(* Logix 5000 AddOnInstructionDefinition export CFW900_2070; software revision 20.06 *)

ADD_ON_INSTRUCTION CFW900_2070   (* revision 1.0, ExecutePrescan *)
// 20/70 CIP Basic Speed
// AOI
// Help:
// Drive setup as follows:
// C9.5.1 = 20/70
// C4.1.1 - Remote 2
// C4.2.2.1 - Ethernet
// C4.2.2.2 - Ethernet
// C4.2.2.3 - Ethernet
// C4.2.2.4 - Ethernet
// C4.3.1.2.1 - Keypad
// C4.3.1.2.2 - Ethernet
VAR_INPUT
   ConnectionFaulted : BOOL; {required}   // From CFW900
END_VAR
VAR_IN_OUT
   InputData : INT[2]; {required}   // Input Assembly From CFW900
   OutputData : INT[2]; {required}   // Output Assembly To CFW900
END_VAR
VAR_INPUT
   Run : BOOL; {visible}   // 1 = Run 0 = Stop
   Fault_Reset : BOOL; {visible}   // 1 = Clear fault 0 = no action
   cfg_FailToStartDelay : DINT; {visible}   // Time in seconds before faulting on fail to start if vfd doesn't start on command (0 to disable)
   cfg_FailToStopDelay : DINT; {visible}   // Time in seconds before faulting on fail to stop if vfd doesn't stop on command (0 to disable)
END_VAR
VAR_OUTPUT
   Connection_Ready : BOOL; {access Read Only, visible}   // 1 = Connection to VFD is established to PLC
   Connection_Faulted : BOOL; {access Read Only, visible}   // Connection_Faulted Status Bit
   Running : BOOL; {access Read Only, visible}   // 1 = CFW900 Running 0 = CFW900 Stopped
   Faulted : BOOL; {access Read Only, visible}   // AOI Faulted Connection fault or failed to start / stop as well as VFD faults
END_VAR
VAR_INPUT
   Speed_Reference : INT; {required}   // Speed Setpoint (RPM) Negative speed will reverse direction
END_VAR
VAR_OUTPUT
   RealSpeed : INT; {access Read Only, visible}   // Current Speed (RPM)
END_VAR
VAR
   FailToStart : TIMER; {access None}
   FailToStop : TIMER;
   Wrk_Run1 : BOOL; {access None}
END_VAR

ROUTINE Logic   (* ladder *)
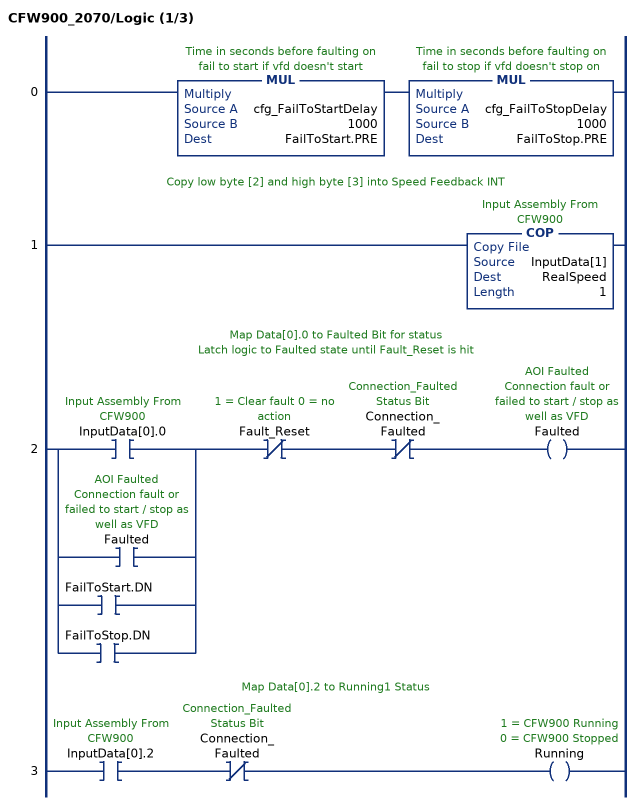
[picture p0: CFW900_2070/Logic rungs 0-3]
   0: MUL(cfg_FailToStartDelay,1000,FailToStart.PRE)MUL(cfg_FailToStopDelay,1000,FailToStop.PRE);
   // Copy low byte [2] and high byte [3] into Speed Feedback INT
   1: COP(InputData[1],RealSpeed,1);
   // Map Data[0].0 to Faulted Bit for status
   // Latch logic to Faulted state until Fault_Reset is hit
   2: [XIC(InputData[0].0) ,XIC(Faulted) ,XIC(FailToStart.DN) ,XIC(FailToStop.DN) ]XIO(Fault_Reset)XIO(Connection_Faulted)OTE(Faulted);
   // Map Data[0].2 to Running1 Status
   3: XIC(InputData[0].2)XIO(Connection_Faulted)OTE(Running);
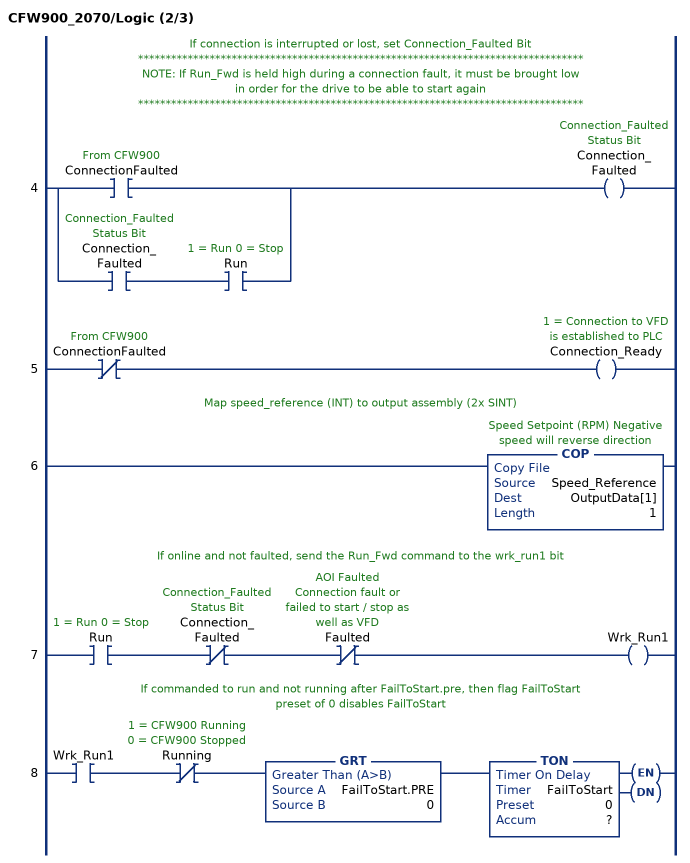
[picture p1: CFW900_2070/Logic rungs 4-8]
   // If connection is interrupted or lost, set Connection_Faulted Bit
   // *********************************************************************************
   // NOTE: If Run_Fwd is held high during a connection fault, it must be brought low
   // in order for the drive to be able to start again
   // *********************************************************************************
   4: [XIC(ConnectionFaulted) ,XIC(Connection_Faulted) XIC(Run) ]OTE(Connection_Faulted);
   5: XIO(ConnectionFaulted)OTE(Connection_Ready);
   // Map speed_reference (INT) to output assembly (2x SINT)
   6: COP(Speed_Reference,OutputData[1],1);
   // If online and not faulted, send the Run_Fwd command to the wrk_run1 bit
   7: XIC(Run)XIO(Connection_Faulted)XIO(Faulted)OTE(Wrk_Run1);
   // If commanded to run and not running after FailToStart.pre, then flag FailToStart
   // preset of 0 disables FailToStart
   8: XIC(Wrk_Run1)XIO(Running)GRT(FailToStart.PRE,0)TON(FailToStart,?,?);
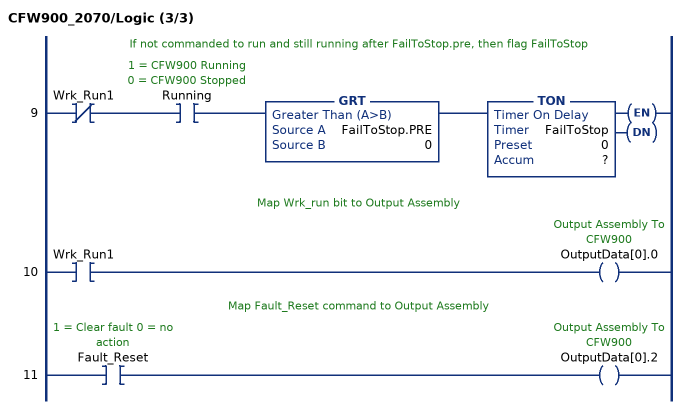
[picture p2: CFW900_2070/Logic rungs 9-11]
   // If not commanded to run and still running after FailToStop.pre, then flag FailToStop
   9: XIO(Wrk_Run1)XIC(Running)GRT(FailToStop.PRE,0)TON(FailToStop,?,?);
   // Map Wrk_run bit to Output Assembly
   10: XIC(Wrk_Run1)OTE(OutputData[0].0);
   // Map Fault_Reset command to Output Assembly
   11: XIC(Fault_Reset)OTE(OutputData[0].2);
END_ROUTINE

ROUTINE Prescan   (* ladder *)
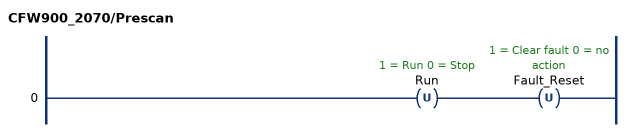
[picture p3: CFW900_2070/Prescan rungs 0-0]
   0: OTU(Run)OTU(Fault_Reset);
END_ROUTINE
END_ADD_ON_INSTRUCTION
